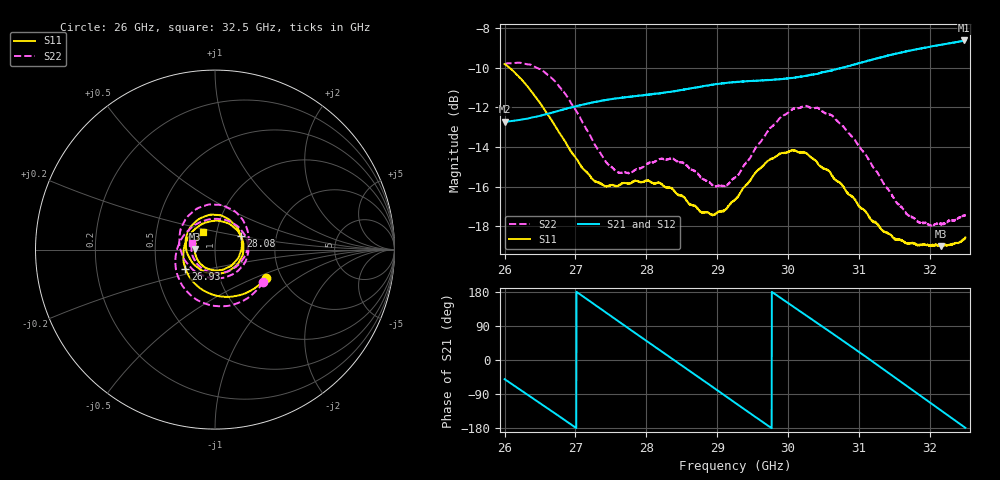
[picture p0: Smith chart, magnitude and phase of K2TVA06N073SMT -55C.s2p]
!Keysight Technologies,N5247B,US57180393,A.17.35.14
!Date: Thursday, May 08, 2025 10:30:43
!Correction: S11(C  2-Port  )
!S21(C  2-Port  )
!S12(C  2-Port  )
!S22(C  2-Port  )
!S2P File: Measurements: S11, S21, S12, S22:
# Hz S  RI  R 50
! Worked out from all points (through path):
!   2001 points, 26 GHz to 32.5 GHz, reference 50 ohm
!   highest |S21| = -8.61 dB at 32.48 GHz (marker M1); lowest = -12.7 dB at 26 GHz (marker M2)
!   lowest |S11| = -19.0 dB at 32.16 GHz (marker M3), VSWR 1.25, Z = 39.9 + j0.284 ohm
!   |S11| at or under -10 dB: 26.07 GHz to end of sweep
!   |S22| runs from -18.0 to -9.7 dB; largest |S21 - S12| = 0.0013
!   S11 on the Smith chart (normalised r, x): 26 GHz: 1.66, -0.58; 26.93 GHz: 0.70, -0.15; 28.08 GHz: 1.31, +0.21; 32.5 GHz: 0.86, +0.17
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2.6e10  0.2829 -0.1563  0.1465 -0.1787  0.1468 -0.1786  0.2676 -0.1813
2.6468e10  0.0293 -0.2608  -0.0809 -0.2245  -0.0807 -0.2245  0.0154 -0.3152
2.69295e10  -0.1644 -0.1058  -0.2466 -0.0471  -0.2466 -0.0476  -0.2005 -0.1643
2.70855e10  -0.1761 -0.024  -0.2515 0.0424  -0.2512 0.042  -0.2206 -0.0746
2.7612e10  -0.0209 0.1581  -0.0519 0.2599  -0.0519 0.2601  -0.0637 0.1593
2.808325e10  0.1428 0.0766  0.2086 0.1735  0.2089 0.1737  0.1466 0.1087
2.816775e10  0.1561 0.0445  0.2387 0.131  0.2392 0.1312  0.1687 0.076
2.8639e10  0.0868 -0.1128  0.2369 -0.1512  0.2373 -0.1508  0.1354 -0.1108
2.896075e10  -0.0377 -0.1293  0.076 -0.2773  0.0761 -0.2764  -2.83e-05 -0.159
2.925e10  -0.1335 -0.0619  -0.1123 -0.2682  -0.1122 -0.269  -0.1286 -0.1066
2.9536e10  -0.1631 0.0526  -0.2542 -0.1466  -0.2541 -0.1465  -0.1972 0.0169
2.97895e10  -0.1214 0.1425  -0.295 0.0142  -0.2951 0.0143  -0.1829 0.1335
3.004625e10  -0.035 0.1924  -0.2417 0.1741  -0.2422 0.1742  -0.1092 0.2224
3.03355e10  0.0659 0.175  -0.0899 0.2903  -0.0898 0.2905  0.00672 0.2501
3.06475e10  0.1356 0.0954  0.1226 0.2882  0.1223 0.2882  0.123 0.2027
3.09725e10  0.1433 -0.0114  0.2946 0.1352  0.2945 0.1355  0.1853 0.0848
3.12e10  0.1042 -0.0757  0.3307 -0.0309  0.3311 -0.0303  0.1769 -0.00959
3.141775e10  0.0453 -0.1115  0.2815 -0.1909  0.2814 -0.1909  0.1304 -0.0842
3.18045e10  -0.0683 -0.0902  0.0256 -0.3515  0.026 -0.3515  -0.00512 -0.1304
3.215875e10  -0.112 0.00351  -0.248 -0.263  -0.2483 -0.2636  -0.1074 -0.0686
3.247725e10  -0.0728 0.0911  -0.37 -0.0259  -0.3693 -0.0262  -0.1302 0.0315
3.25e10  -0.0683 0.096  -0.3707 -0.00664  -0.3712 -0.00649  -0.1281 0.0388
